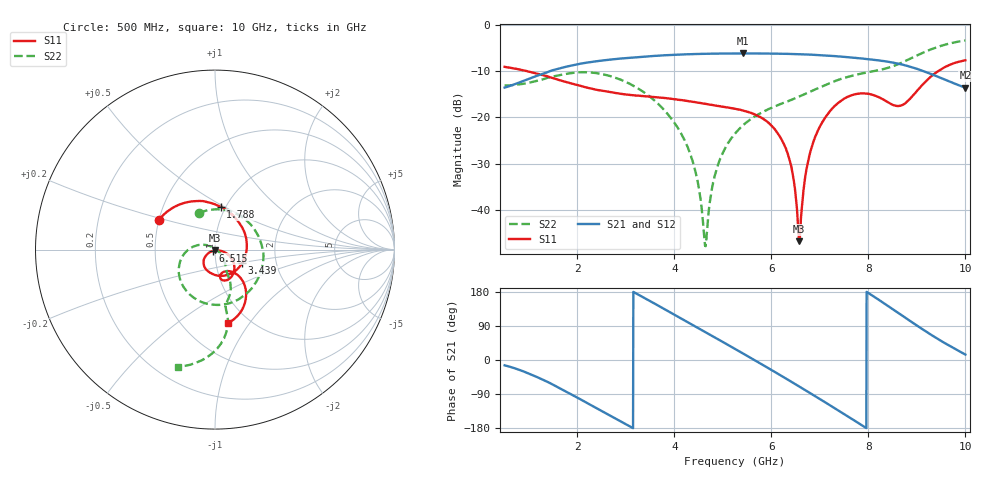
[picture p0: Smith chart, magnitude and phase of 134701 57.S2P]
!  2-Port S-parameters saved by WinCal
! VAR MeasName=S-Parameters (CALIBRATED_DATA) read from VNA (N5242A)
! VAR MeasDate=2013-7-3 16:40:44
! VAR NAME=134701 57
! VAR FILENAME=134701 57.S2P
! VAR DATE=2013-7-3 16:40:44
! VAR PHYS_PORTS=1,2
# Hz S MA R 50
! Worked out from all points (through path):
!   1601 points, 500 MHz to 10 GHz, reference 50 ohm
!   highest |S21| = -6.12 dB at 5.422 GHz (marker M1); lowest = -13.5 dB at 10 GHz (marker M2)
!   lowest |S11| = -46.8 dB at 6.574 GHz (marker M3), VSWR 1.01, Z = 50 - j0.457 ohm
!   |S11| at or under -10 dB: 978.2 MHz to 9.434 GHz (8.455 GHz wide, 162 % of centre)
!   |S22| runs from -47.9 to -3.3 dB; largest |S21 - S12| = 0.002
!   S11 on the Smith chart (normalised r, x): 500 MHz: 0.50, +0.19; 1.788 GHz: 0.95, +0.48; 3.439 GHz: 1.34, -0.21; 6.515 GHz: 0.98, -0.01; 10 GHz: 0.80, -0.79
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5e8  0.3537 152.1  0.2107 -14.0  0.2102 -13.9  0.222 113.5
1.23625e9  0.2923 112.5  0.2915 -48.9  0.2918 -48.9  0.2546 14.8
1.788438e9  0.2409 82.6  0.3567 -84.8  0.3569 -84.8  0.2981 -48.1
2.085312e9  0.2188 65.5  0.3844 -105.3  0.3845 -105.4  0.3096 -76.6
2.768125e9  0.1849 20.7  0.4285 -153.3  0.4282 -153.3  0.2717 -130.5
3.439062e9  0.1691 -26.9  0.4591 159.7  0.4593 159.7  0.1772 -171.0
3.670625e9  0.1653 -42.3  0.4682 143.3  0.4677 143.3  0.1397 177.3
4.317812e9  0.1496 -78.0  0.485 96.9  0.4854 97.0  0.04136 147.6
4.484062e9  0.1452 -85.0  0.4869 84.9  0.4883 84.9  0.01971 134.6
4.638438e9  0.1408 -91.0  0.49 73.8  0.4901 73.8  0.004221 50.8
4.87e9  0.1339 -98.8  0.4919 56.9  0.4927 56.9  0.02723 -33.1
5.25e9  0.1243 -110.5  0.4938 29.3  0.4941 29.2  0.06705 -46.7
5.422188e9  0.1186 -116.2  0.4945 16.7  0.4941 16.6  0.0827 -51.0
6.2e9  0.05896 -146.8  0.4904 -41.3  0.4904 -41.3  0.1407 -62.1
6.401875e9  0.03043 -153.5  0.4885 -56.6  0.4886 -56.7  0.1546 -63.1
6.514688e9  0.01206 -146.5  0.4862 -65.3  0.4868 -65.5  0.1637 -63.5
6.574062e9  0.004572 -88.4  0.4844 -70.0  0.485 -70.1  0.1688 -63.5
6.835312e9  0.04848 -13.3  0.4788 -90.3  0.479 -90.2  0.1937 -64.8
7.53e9  0.163 -49.9  0.4517 -145.2  0.4527 -145.2  0.2708 -72.8
8.420625e9  0.1447 -78.1  0.4006 141.2  0.3998 141.1  0.3471 -79.5
8.996562e9  0.1927 -48.2  0.3373 91.3  0.3372 91.2  0.468 -82.4
1e10  0.4163 -80.3  0.2105 14.3  0.2107 14.2  0.6832 -107.4
